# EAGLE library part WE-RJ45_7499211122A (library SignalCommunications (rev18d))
Order Code 7499211122A Design THT xBase-T 10/100 Base-T PoE Ports 1x1 Application PoE Tab Position DOWN LED (Left-Right) YELLOW-GREEN EMI Fingers Yes Details see: http://katalog.we-online.de/en/pbs/WE-LAN_RJ45/7499211122A? Updated by Yingchun Shan 2016-08-30 2016(C) Würth Elektronik
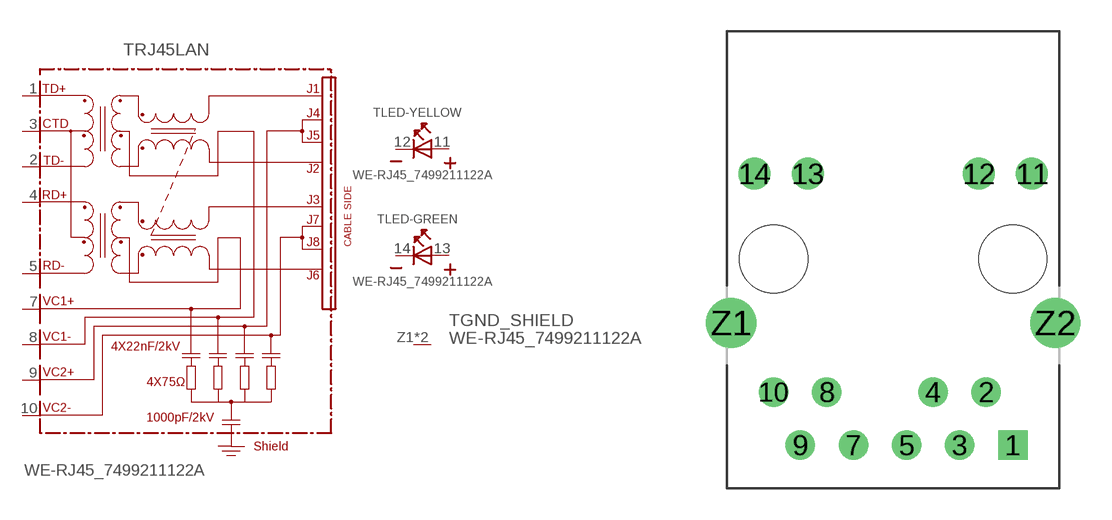
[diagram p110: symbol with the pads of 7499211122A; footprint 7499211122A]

Designator prefix T; gates RJ45LAN=749921-TYPE-2 LED-YELLOW=LED2PIN LED-GREEN=LED2PIN GND_SHIELD=GNDPIN

## WE-RJ45_7499211122A (COMPANY-URL: http://www.we-online.de; CREATED-BY: Christin Zierenner; CREATED-DATE: AUG 2012; DATASHEET-URL: http://katalog.we-online.de/kataloge/eisos/media/pdf/7499211122A.pdf; MANUFACTURER: Würth Elektronik eiSos GmbH)  [7499211122A]
1  RJ45LAN:TD+
2  RJ45LAN:TD-
3  RJ45LAN:CTD
4  RJ45LAN:RD+
5  RJ45LAN:RD-
7  RJ45LAN:VC1+  pwr
8  RJ45LAN:VC1-  pwr
9  RJ45LAN:VC2+  pwr
10  RJ45LAN:VC2-  pwr
11  LED-YELLOW:A  pas
12  LED-YELLOW:K  pas
13  LED-GREEN:A  pas
14  LED-GREEN:K  pas
Z1  GND_SHIELD:GND  pwr
Z2  GND_SHIELD:GND  pwr

## Footprint 7499211122A (pad centres in mm)
MAX HEIGHT=13.74mm PORTS----1X1 LED --YES
drill 0.9 square: 1 5.715,-8.89
drill 0.9: 2 4.445,-6.35; 3 3.175,-8.89; 4 1.905,-6.35; 5 0.635,-8.89; 7 -1.905,-8.89; 8 -3.175,-6.35; 9 -4.445,-8.89; 10 -5.715,-6.35
drill 1.02: 11 6.63,4.08; 12 4.09,4.08; 13 -4.09,4.08; 14 -6.63,4.08
drill 1.6: Z1 -7.745,-3.05; Z2 7.745,-3.05
hole 3.25 at 5.715,0
hole 3.25 at -5.715,0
